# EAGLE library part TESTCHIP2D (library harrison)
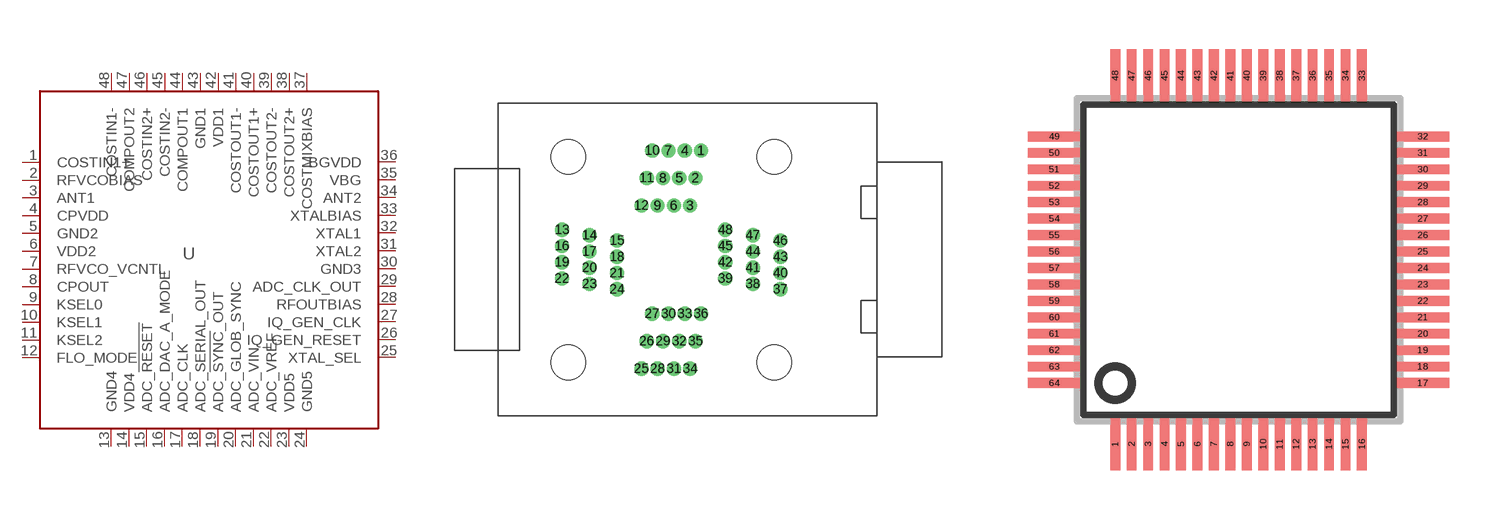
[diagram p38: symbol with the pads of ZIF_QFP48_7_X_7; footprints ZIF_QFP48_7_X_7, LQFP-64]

Designator prefix U

## TESTCHIP2DZIF  [ZIF_QFP48_7_X_7]
1  COSTIN1+
2  RFVCOBIAS
3  ANT1
4  CPVDD
5  GND2
6  VDD2
7  RFVCO_VCNTL
8  CPOUT
9  KSEL0
10  KSEL1
11  KSEL2
12  FLO_MODE
13  GND4
14  VDD4
15  ADC_!RESET!
16  ADC_DAC_A_MODE
17  ADC_CLK
18  ADC_SERIAL_OUT
19  ADC_!SYNC!_OUT
20  ADC_GLOB_SYNC
21  ADC_VIN
22  ADC_VREF
23  VDD5
24  GND5
25  XTAL_SEL
26  IQ_GEN_RESET
27  IQ_GEN_CLK
28  RFOUTBIAS
29  ADC_CLK_OUT
30  GND3
31  XTAL2
32  XTAL1
33  XTALBIAS
34  ANT2
35  VBG
36  BGVDD
37  COSTMIXBIAS
38  COSTOUT2+
39  COSTOUT2-
40  COSTOUT1+
41  COSTOUT1-
42  VDD1
43  GND1
44  COMPOUT1
45  COSTIN2-
46  COSTIN2+
47  COMPOUT2
48  COSTIN1-

## TESTCHIP2DQFP  [LQFP-64]
Pads as for ZIF_QFP48_7_X_7

## Footprint ZIF_QFP48_7_X_7 (pad centres in mm)
drill 0.8 pad 1.27: 1 2.75,10.08; 2 2.25,7.54; 3 1.75,5; 4 1.25,10.08; 5 0.75,7.54; 6 0.25,5; 7 -0.25,10.08; 8 -0.75,7.54; 9 -1.25,5; 10 -1.75,10.08; 11 -2.25,7.54; 12 -2.75,5; 13 -10.08,2.75; 14 -7.54,2.25; 15 -5,1.75; 16 -10.08,1.25; 17 -7.54,0.75; 18 -5,0.25; 19 -10.08,-0.25; 20 -7.54,-0.75; 21 -5,-1.25; 22 -10.08,-1.75; 23 -7.54,-2.25; 24 -5,-2.75; 25 -2.75,-10.08; 26 -2.25,-7.54; 27 -1.75,-5; 28 -1.25,-10.08; 29 -0.75,-7.54; 30 -0.25,-5; 31 0.25,-10.08; 32 0.75,-7.54; 33 1.25,-5; 34 1.75,-10.08; 35 2.25,-7.54; 36 2.75,-5; 37 10.08,-2.75; 38 7.54,-2.25; 39 5,-1.75; 40 10.08,-1.25; 41 7.54,-0.75; 42 5,-0.25; 43 10.08,0.25; 44 7.54,0.75; 45 5,1.25; 46 10.08,1.75; 47 7.54,2.25; 48 5,2.75
hole 3.2 at 9.5,9.5
hole 3.2 at -9.5,9.5
hole 3.2 at -9.5,-9.5
hole 3.2 at 9.5,-9.5

## Footprint LQFP-64 (pad centres in mm)
smd 0.3 x 1.6: 1 -3.75,-5.6; 2 -3.25,-5.6; 3 -2.75,-5.6; 4 -2.25,-5.6; 5 -1.75,-5.6; 6 -1.25,-5.6; 7 -0.75,-5.6; 8 -0.25,-5.6; 9 0.25,-5.6; 10 0.75,-5.6; 11 1.25,-5.6; 12 1.75,-5.6; 13 2.25,-5.6; 14 2.75,-5.6; 15 3.25,-5.6; 16 3.75,-5.6; 33 3.75,5.6; 34 3.25,5.6; 35 2.75,5.6; 36 2.25,5.6; 37 1.75,5.6; 38 1.25,5.6; 39 0.75,5.6; 40 0.25,5.6; 41 -0.25,5.6; 42 -0.75,5.6; 43 -1.25,5.6; 44 -1.75,5.6; 45 -2.25,5.6; 46 -2.75,5.6; 47 -3.25,5.6; 48 -3.75,5.6
smd 1.6 x 0.3: 17 5.6,-3.75; 18 5.6,-3.25; 19 5.6,-2.75; 20 5.6,-2.25; 21 5.6,-1.75; 22 5.6,-1.25; 23 5.6,-0.75; 24 5.6,-0.25; 25 5.6,0.25; 26 5.6,0.75; 27 5.6,1.25; 28 5.6,1.75; 29 5.6,2.25; 30 5.6,2.75; 31 5.6,3.25; 32 5.6,3.75; 49 -5.6,3.75; 50 -5.6,3.25; 51 -5.6,2.75; 52 -5.6,2.25; 53 -5.6,1.75; 54 -5.6,1.25; 55 -5.6,0.75; 56 -5.6,0.25; 57 -5.6,-0.25; 58 -5.6,-0.75; 59 -5.6,-1.25; 60 -5.6,-1.75; 61 -5.6,-2.25; 62 -5.6,-2.75; 63 -5.6,-3.25; 64 -5.6,-3.75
